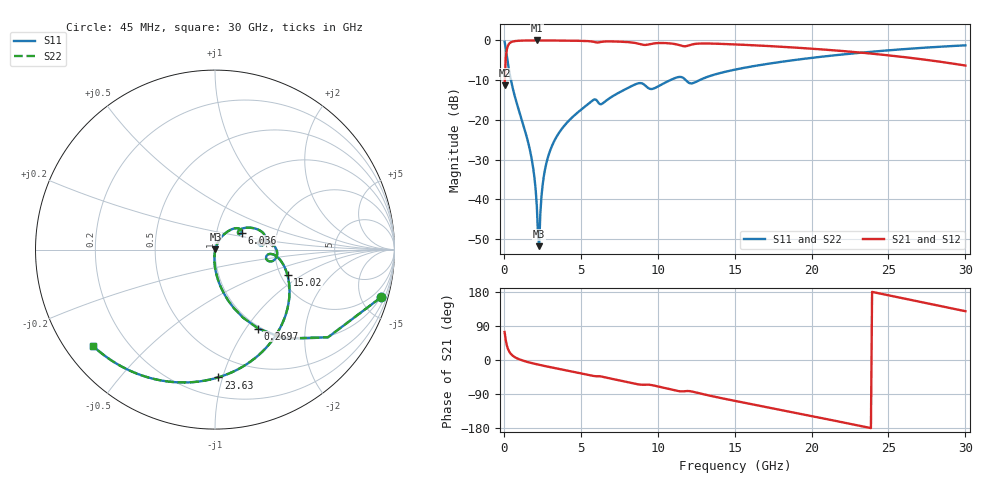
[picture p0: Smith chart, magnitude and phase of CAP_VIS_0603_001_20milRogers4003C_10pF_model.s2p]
! S-parameter model data by Modelithics Inc.  support@modelithics.com  813-866-6335  Tampa FL USA
! S-Parameter data specifications:
! Substrate: 20-mil Rogers 4003C, substrate thickness, H=0.508mm, Dielectric constant, Er=3.75
! PCB Mounting Pad Footprint: Pad width, PadW=0.90mm , Pad length, PadL=1.00mm , Pad gap, PadG (edge-to-edge)=1.00mm , Reference planes=3.0mm apart
! Created Wed Nov 18 13:25:45 2015
# hz S ma R 50
! 2 Port Network Data from SP1.SP block
! freq  magS11  angS11  magS21  angS21  magS12  angS12  magS22  angS22
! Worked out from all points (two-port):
!   401 points, 45 MHz to 30 GHz, reference 50 ohm
!   highest |S21| = -0.02 dB at 2.142 GHz (marker M1); lowest = -11.3 dB at 45 MHz (marker M2)
!   |S21| within 3 dB of the highest: 166.4 MHz to 23.04 GHz (22.87 GHz wide, 197 % of centre)
!   lowest |S11| = -51.8 dB at 2.292 GHz (marker M3), VSWR 1.01, Z = 50.2 + j0.124 ohm
!   |S11| at or under -10 dB: 457.4 MHz to 10.81 GHz (10.36 GHz wide, 184 % of centre); 11.82 GHz to 12.71 GHz (887 MHz wide, 7.23 % of centre)
!   |S22| runs from -51.8 to -0.3 dB; largest |S21 - S12| = 0
!   S11 on the Smith chart (normalised r, x): 45 MHz: 0.97, -6.94; 269.7 MHz: 0.97, -1.14; 6.036 GHz: 1.32, +0.26; 15.02 GHz: 2.17, -0.76; 23.63 GHz: 0.33, -0.97; 30 GHz: 0.08, -0.34
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4.5e7  0.962 -16.1  0.273 73.9  0.273 73.9  0.962 -16.1
2.696625e8  0.5015 -61.3  0.8645 28.6  0.8645 28.6  0.5015 -61.3
4.194375e8  0.343 -72.1  0.9385 17.8  0.9385 17.8  0.343 -72.1
6.441e8  0.2208 -80.5  0.9742 9.2  0.9742 9.2  0.2208 -80.5
1.767412e9  0.03534 -94.9  0.9975 -7.7  0.9975 -7.7  0.03534 -94.9
1.992075e9  0.01825 -94.2  0.9979 -9.9  0.9979 -9.9  0.01825 -94.2
2.14185e9  0.008099 -87.9  0.9979 -11.3  0.9979 -11.3  0.008099 -87.9
2.291625e9  0.002585 28.6  0.9979 -12.7  0.9979 -12.7  0.002585 28.6
2.366512e9  0.006582 59.2  0.9978 -13.3  0.9978 -13.3  0.006582 59.2
2.516288e9  0.01519 67.6  0.9976 -14.7  0.9976 -14.7  0.01519 67.6
2.666062e9  0.02351 68.9  0.9974 -16.0  0.9974 -16.0  0.02351 68.9
3.0405e9  0.04298 67.8  0.9965 -19.1  0.9965 -19.1  0.04298 67.8
3.789375e9  0.07839 62.8  0.9939 -25.3  0.9939 -25.3  0.07839 62.8
5.062462e9  0.1367 52.5  0.9855 -35.6  0.9855 -35.6  0.1367 52.5
6.036e9  0.1759 32.7  0.9409 -42.8  0.9409 -42.8  0.1759 32.7
8.73195e9  0.2883 16.3  0.911 -64.3  0.911 -64.3  0.2883 16.3
1.007992e10  0.2675 11.5  0.9262 -70.5  0.9262 -70.5  0.2675 11.5
1.50225e10  0.4288 -19.5  0.8897 -107.9  0.8897 -107.9  0.4288 -19.5
2.003996e10  0.6037 -59.2  0.7856 -148.3  0.7856 -148.3  0.6037 -59.2
2.363456e10  0.7123 -88.6  0.6893 -177.8  0.6893 -177.8  0.7123 -88.6
2.505742e10  0.7515 -100.4  0.6465 170.3  0.6465 170.3  0.7515 -100.4
3e10  0.8666 -141.9  0.4827 128.8  0.4827 128.8  0.8666 -141.9
